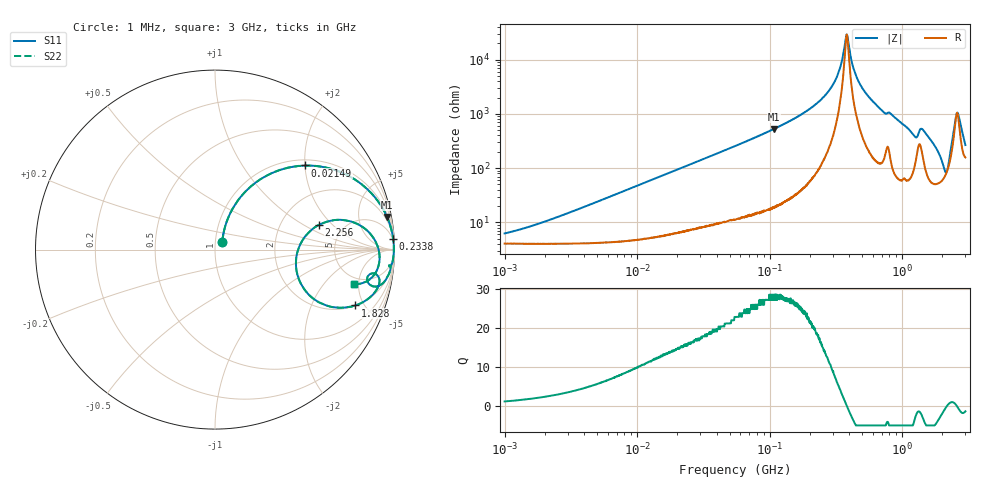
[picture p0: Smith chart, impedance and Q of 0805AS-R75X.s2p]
!s-Parameter Generated by FASTRON Sdn. Bhd.
!FASTRON P/N : 0805AS-R75X
!Keysight Technologies: E4991B_MY54100416_A.01.15
!Date: Mon Jun 15 12:55:59 2026
!Version  :Rev01  Mon Jun 15 12:55:59 2026
!Data & Calibration Information:
!Freq  S11  S21  S12  S22
!PortZ  Port1:50+j0  Port2:50+j0
!When reading reference impedance value at option line is always used.
! Remarks : This data is being provided solely for informational purposes.
# Hz S dB R 50
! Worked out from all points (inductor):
!   1601 points, 1 MHz to 3 GHz, reference 50 ohm
!   read as one part in series: L = 755 nH near 2.562 MHz
!   highest Q = 28.5 at 107.1 MHz (marker M1), where L = 778 nH
!   self-resonance near 381.7 MHz
!   S11 on the Smith chart (normalised r, x): 1 MHz: 1.08, +0.10; 21.49 MHz: 1.13, +2.01; 233.8 MHz: 3, +33; 1.828 GHz: 2.02, -4.31; 2.256 GHz: 3.29, +1.41; 3 GHz: 4.15, -4.32
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1000000  -24.40 46.9  -0.35 -2.6  -0.35 -2.6  -24.40 46.9
3804036  -15.10 67.4  -0.48 -9.8  -0.48 -9.8  -15.10 67.4
1.447069e7  -5.29 52.6  -1.97 -32.8  -1.97 -32.8  -5.29 52.6
2.148682e7  -3.26 43.0  -3.31 -43.3  -3.31 -43.3  -3.26 43.0
5.504702e7  -0.74 21.0  -8.92 -66.5  -8.92 -66.5  -0.74 21.0
1.070951e8  -0.21 10.7  -14.60 -77.2  -14.60 -77.2  -0.21 10.7
2.083556e8  -0.06 4.3  -22.50 -83.0  -22.50 -83.0  -0.06 4.3
2.3377e8  -0.05 3.4  -24.50 -83.3  -24.50 -83.3  -0.05 3.4
3.156319e8  -0.03 1.3  -32.80 -80.5  -32.80 -80.5  -0.03 1.3
3.817355e8  -0.03 0.0  -49.30 -1.3  -49.30 -1.3  -0.03 0.0
4.32606e8  -0.03 -0.9  -36.30 75.2  -36.30 75.2  -0.03 -0.9
4.853736e8  -0.04 -1.7  -30.60 80.4  -30.60 80.4  -0.04 -1.7
6.685918e8  -0.09 -4.3  -22.40 80.3  -22.40 80.3  -0.09 -4.3
7.925923e8  -0.20 -5.2  -20.70 72.9  -20.70 72.9  -0.20 -5.2
1.237271e9  -0.80 -13.0  -12.60 61.6  -12.60 61.6  -0.80 -13.0
1.423359e9  -0.67 -9.7  -15.00 60.8  -15.00 60.8  -0.67 -9.7
1.827992e9  -1.50 -21.7  -8.40 54.9  -8.40 54.9  -1.50 -21.7
1.990301e9  -3.31 -26.7  -6.08 38.2  -6.08 38.2  -3.31 -26.7
2.113475e9  -6.33 -17.4  -5.06 15.0  -5.06 15.0  -6.33 -17.4
2.255531e9  -4.50 13.4  -7.07 -18.1  -7.07 -18.1  -4.50 13.4
2.594767e9  -0.79 -0.4  -21.20 4.1  -21.20 4.1  -0.79 -0.4
3e9  -1.99 -13.9  -10.50 39.9  -10.50 39.9  -1.99 -13.9
